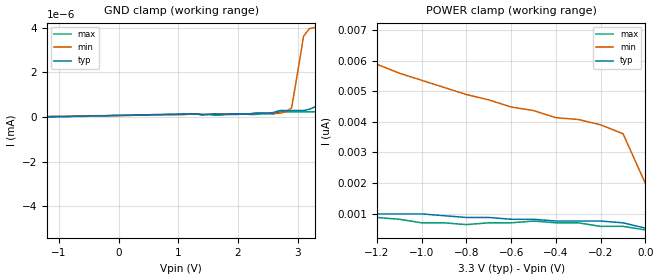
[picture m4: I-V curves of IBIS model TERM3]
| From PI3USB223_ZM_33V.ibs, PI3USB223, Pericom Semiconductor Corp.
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|   Model TERM3
[Model] TERM3
Model_type Terminator
| variable   typ   min   max
C_comp   4.000pF   3.950pF   4.050pF
[Voltage Range]   3.300V   3.000V   3.600V
[GND Clamp Reference]   0.000V   0.000V   0.000V
[POWER Clamp Reference]   3.300V   3.000V   3.600V
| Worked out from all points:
|   GND clamp passes 1 mA (typ) near -2.87 V on its own axis
[GND Clamp]
| Voltage   I(typ)   I(min)   I(max)
-3.3V     -1.252A    -1.714A    -789.2mA
-2.5V     -2.087uA   -12.88uA   -82.31nA
-2.4V     -76.98nA   -966nA     -1.281nA
-2.3V     -2.357nA   -52.88nA   -116.4pA
-2.2V     -145.5pA   -2.445nA   -145.5pA
-2.1V     -145.5pA   -232.8pA   -58.21pA
-1.6V     -58.21pA   0A         -58.21pA
2.8V      291pA      232.8pA    232.8pA
2.9V      291pA      407.5pA    232.8pA
3.1V      291pA      3.609nA    232.8pA
3.2V      349.2pA    3.958nA    232.8pA
3.3V      465.7pA    4.016nA    232.8pA
[POWER Clamp]   |Note: Vtable = Vcc - Voutput
| Voltage   I(typ)   I(min)   I(max)
-3.3V     1.863nA    21.89nA    1.048nA
-2.8V     1.397nA    15.13nA    931.3pA
-2.7V     1.513nA    14.2nA     1.048nA
-2.2V     1.164nA    10.19nA    931.3pA
-2.1V     1.164nA    9.488nA    698.5pA
-2V       1.164nA    8.964nA    931.3pA
-1.7V     1.164nA    7.509nA    698.5pA
-1.6V     1.048nA    7.101nA    873.1pA
-800mV    873.1pA    4.889nA    640.3pA
-500mV    814.9pA    4.366nA    756.7pA
-100mV    698.5pA    3.609nA    582.1pA
0V        523.9pA    1.979nA    465.7pA
